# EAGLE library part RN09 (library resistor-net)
RESISTOR NETWORK
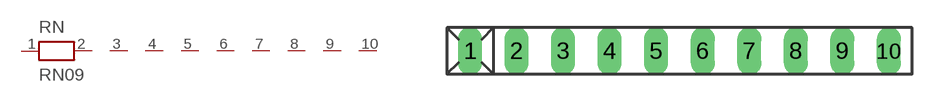
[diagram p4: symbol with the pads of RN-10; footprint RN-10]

Designator prefix RN

## RN09 (OC_FARNELL: unknown; OC_NEWARK: unknown)  [RN-10]
1  1  pas
2  2  pas
3  3  pas
4  4  pas
5  5  pas
6  6  pas
7  7  pas
8  8  pas
9  9  pas
10  10  pas

## Footprint RN-10 (pad centres in mm)
RESISTOR NETWORK
drill 0.813 long: 1 -11.43,0; 2 -8.89,0; 3 -6.35,0; 4 -3.81,0; 5 -1.27,0; 6 1.27,0; 7 3.81,0; 8 6.35,0; 9 8.89,0; 10 11.43,0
